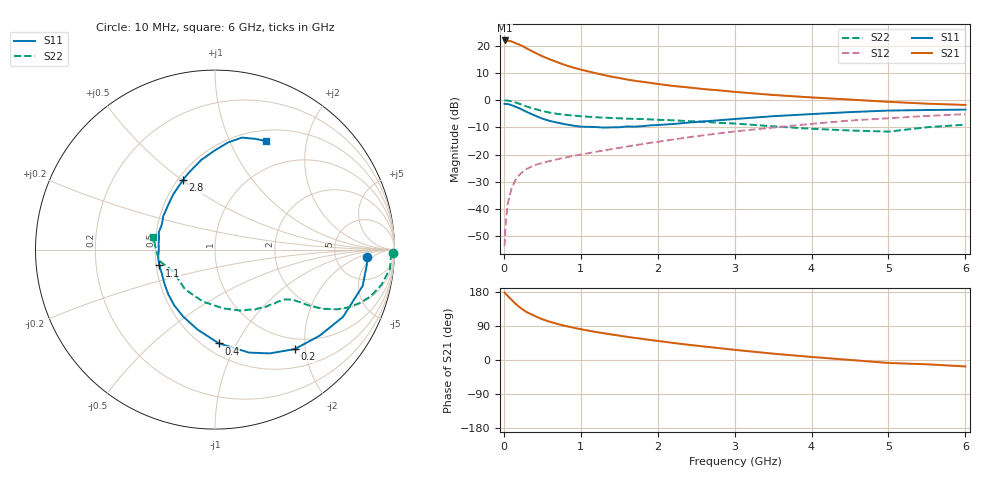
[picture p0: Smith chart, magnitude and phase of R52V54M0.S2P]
! SIEMENS Small Signal Semiconductors
! BFR183
! Si NPN RF Bipolar Junction Transistor in SOT23
! VCE = 2.5 V  IC = 4 mA
! Common Emitter S-Parameters:  May  1996
# GHz  S  MA  R  50
!  f  S11  S21  S12  S22
! GHz  MAG  ANG  MAG  ANG  MAG  ANG  MAG  ANG
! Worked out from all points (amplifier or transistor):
!   36 points, 10 MHz to 6 GHz, reference 50 ohm
!   highest |S21| = 21.8 dB at 10 MHz (marker M1)
!   |S21| within 3 dB of that: start of sweep to 301.5 MHz
!   unconditionally stable (mu >= 1): 1.129 GHz to 2.68 GHz
!   at 250 MHz: K = 0.36, MSG = 22.9 dB, |S12| = -26.2 dB
!   at 1.4 GHz: K = 1.06, MAG = 11.8 dB, |S12| = -18.0 dB
!   at 6 GHz: K = 0.89, MSG = 1.7 dB, |S12| = -5.2 dB
!   S11 on the Smith chart (normalised r, x): 10 MHz: 11, -3; 200 MHz: 0.80, -1.80; 400 MHz: 0.59, -0.85; 1.1 GHz: 0.52, -0.10; 2.8 GHz: 0.53, +0.50; 6 GHz: 0.63, +1.38
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0.01  0.8495 -2.8  12.37 178.0  0.0021 86.4  0.9913 -1.2
0.02  0.85 -5.7  12.25 175.4  0.0047 88.7  0.9811 -2.4
0.05  0.8473 -13.8  12.19 169.2  0.0125 81.8  0.9807 -6.2
0.1  0.8059 -27.7  11.9 158.8  0.024 75.8  0.9482 -11.9
0.15  0.7552 -39.4  11.06 148.7  0.0342 69.7  0.9046 -16.8
0.2  0.7103 -51.3  10.4 140.3  0.0424 65.1  0.8561 -20.5
0.25  0.6537 -62.2  9.612 132.5  0.0488 61.0  0.8039 -23.7
0.3  0.6043 -71.7  8.781 126.2  0.055 58.6  0.7589 -26.0
0.4  0.5231 -87.6  7.44 116.4  0.064 54.5  0.6867 -28.7
0.5  0.4569 -102.1  6.359 107.5  0.0706 53.0  0.6292 -30.3
0.6  0.4132 -115.4  5.561 100.7  0.0767 52.4  0.5871 -31.2
0.7  0.3848 -126.2  4.913 95.0  0.0824 52.4  0.5581 -31.7
0.9  0.3405 -145.7  3.945 85.4  0.0947 52.9  0.5194 -32.7
1.1  0.3228 -164.1  3.343 77.5  0.1061 54.6  0.4941 -34.3
1.4  0.3158 174.0  2.683 67.3  0.1259 55.9  0.4703 -36.9
1.6  0.328 162.7  2.38 61.2  0.1405 56.5  0.4564 -39.3
2.2  0.3641 134.7  1.814 45.1  0.1891 56.0  0.4264 -48.5
2.8  0.4268 114.6  1.505 31.3  0.246 52.7  0.3828 -61.0
3.5  0.5061 98.6  1.24 16.8  0.3136 45.9  0.3304 -82.2
4.5  0.6017 83.0  1.022 0.2  0.4214 34.0  0.2771 -127.2
5.5  0.6568 69.9  0.859 -11.3  0.5115 21.1  0.3175 -168.9
6  0.6683 64.6  0.814 -17.0  0.5518 12.7  0.3545 168.3
